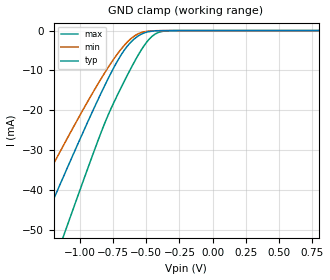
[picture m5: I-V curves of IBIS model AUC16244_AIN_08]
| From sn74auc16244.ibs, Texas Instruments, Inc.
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[Model]   AUC16244_AIN_08
Model_type  Input
Vinl=0
Vinh=0.8
| variable   typ   min   max
C_comp   3.23pF   2.64pF   3.78pF
[Temperature Range]   40   100   -40
| Ambient temperature   25   85   -40
[Voltage range]   0.8   0.8   0.8
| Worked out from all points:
|   GND clamp passes 1 mA (typ) near -0.54 V on its own axis
[GND Clamp]
| AUC16244_AIN_08
|   Voltage   I(typ)   I(min)   I(max)
-3.6V     -231.9mA   -193.8mA   -279.4mA
-1.465V   -62.98mA   -50.31mA   -83.3mA
-1.33V    -52.45mA   -41.66mA   -70.73mA
-1.285V   -48.96mA   -38.8mA    -66.53mA
-1.12V    -36.28mA   -28.5mA    -51.14mA
-1.085V   -33.62mA   -26.35mA   -47.88mA
-830mV    -14.93mA   -11.49mA   -24.63mA
-700mV    -6.66mA    -5.077mA   -14.99mA
-580mV    -1.812mA   -1.157mA   -7.258mA
-450mV    -131uA     -62.06uA   -1.277mA
-315mV    -2.578uA   -1.609uA   -22.45uA
800mV     103.7pA    191.9pA    83.29pA
